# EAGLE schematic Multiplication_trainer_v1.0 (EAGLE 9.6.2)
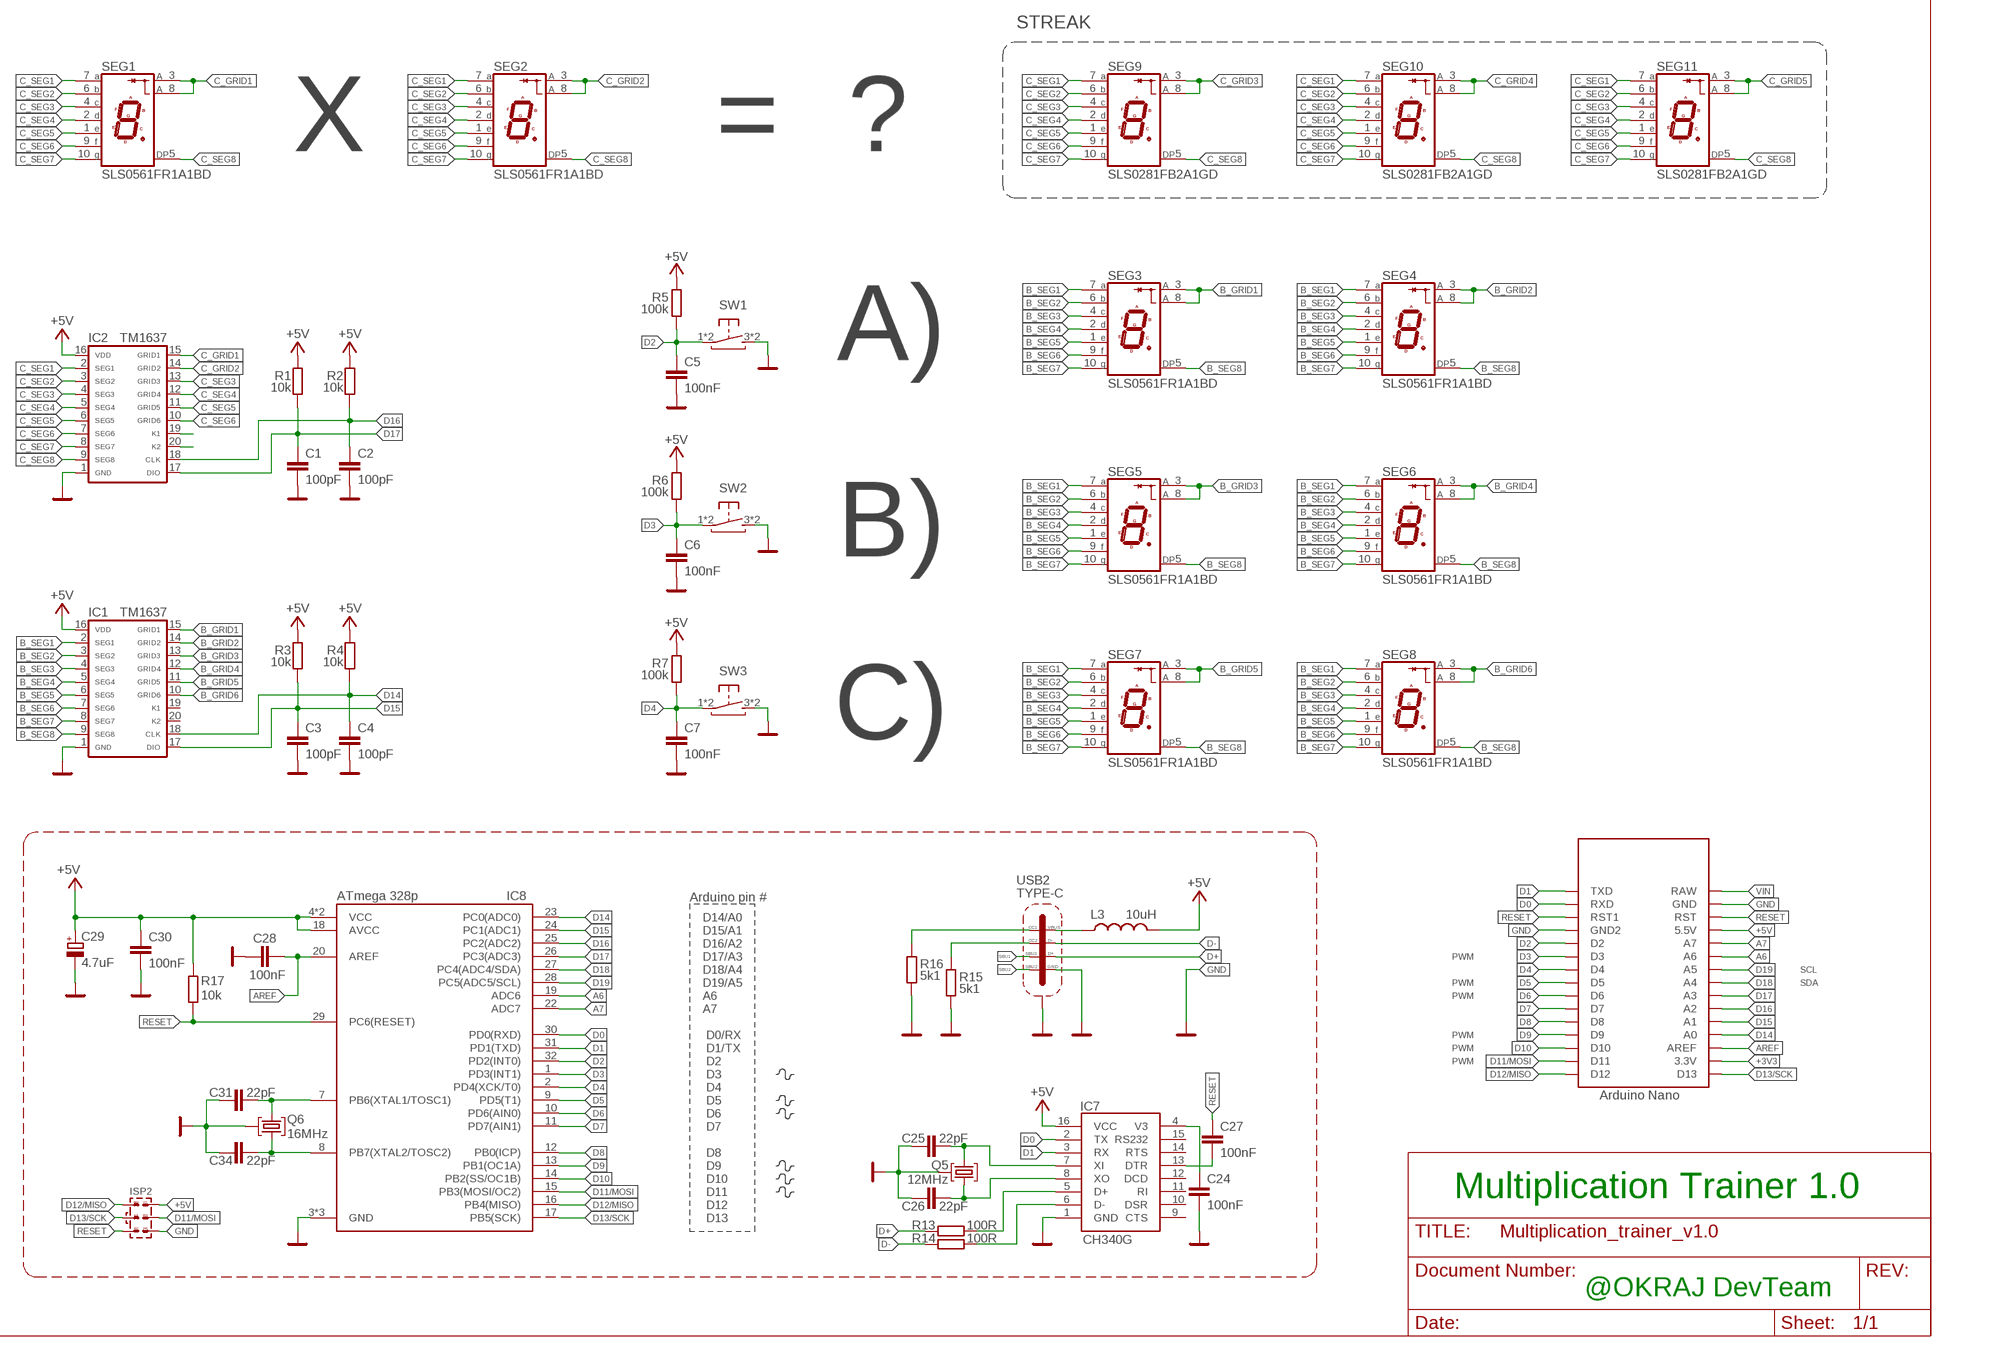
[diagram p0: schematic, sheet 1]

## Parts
C1  100pF  C-EUC0805K  [C0805K]
C2  100pF  C-EUC0805K  [C0805K]
C3  100pF  C-EUC0805K  [C0805K]
C4  100pF  C-EUC0805K  [C0805K]
C5  100nF  C-EUC0805  [C0805]
C6  100nF  C-EUC0805  [C0805]
C7  100nF  C-EUC0805  [C0805]
C24  100nF  C-EUC0603  [C0603]
C25  22pF  C-EUC0603  [C0603]
C26  22pF  C-EUC0603  [C0603]
C27  100nF  C-EUC0603  [C0603]
C28  100nF  C-EUC0603  [C0603]
C29  4.7uF  CPOL-EUSMCA  [SMC_A]
C30  100nF  C-EUC0603  [C0603]
C31  22pF  C-EUC0603  [C0603]
C34  22pF  C-EUC0603  [C0603]
IC1  TM1637  [SOP20]
IC2  TM1637  [SOP20]
IC7  CH340G  CH340GSMD  [SOIC16]
IC8  ATmega 328p  ATMEGA328PQFP32N_ROUND-PADS  [QFP80P900X900X120-32N_ROUND-PADS]
ISP2  AVR-ISP-SPI  [AVR-ISP-SPI]
L3  10uH  L-USL0805  [R0805]
Q5  12MHz  KRYSTAL  [ILCX13-FF5F18-16.0000]
Q6  16MHz  KRYSTAL  [ILCX13-FF5F18-16.0000]
R1  10k  R-EU_R0805  [R0805]
R2  10k  R-EU_R0805  [R0805]
R3  10k  R-EU_R0805  [R0805]
R4  10k  R-EU_R0805  [R0805]
R5  100k  R-EU_R0805  [R0805]
R6  100k  R-EU_R0805  [R0805]
R7  100k  R-EU_R0805  [R0805]
R13  100R  R-EU_R0603  [R0603]
R14  100R  R-EU_R0603  [R0603]
R15  5k1  R-EU_R0603  [R0603]
R16  5k1  R-EU_R0603  [R0603]
R17  10k  R-EU_R0603  [R0603]
SEG1  SLS0561FR1A1BD  [SLS0561FR1A1BD]
SEG2  SLS0561FR1A1BD  [SLS0561FR1A1BD]
SEG3  SLS0561FR1A1BD  [SLS0561FR1A1BD]
SEG4  SLS0561FR1A1BD  [SLS0561FR1A1BD]
SEG5  SLS0561FR1A1BD  [SLS0561FR1A1BD]
SEG6  SLS0561FR1A1BD  [SLS0561FR1A1BD]
SEG7  SLS0561FR1A1BD  [SLS0561FR1A1BD]
SEG8  SLS0561FR1A1BD  [SLS0561FR1A1BD]
SEG9  SLS0281FB2A1GD  [SLS0281FB2A1GD]
SEG10  SLS0281FB2A1GD  [SLS0281FB2A1GD]
SEG11  SLS0281FB2A1GD  [SLS0281FB2A1GD]
SW1  TACT-SW_BTNSMTJLC_6X6X4.5  [TACTSW_6X6X4.5_SMT]
SW2  TACT-SW_BTNSMTJLC_6X6X4.5  [TACTSW_6X6X4.5_SMT]
SW3  TACT-SW_BTNSMTJLC_6X6X4.5  [TACTSW_6X6X4.5_SMT]
U$2  NANOTHT-NOUSB  [NANO-NOUSB]
USB2  TYPE-C  TYPE-C-31-M-12TYPE-C-31_L8.94_W7.3  [TYPE-C-31_L8.94_W7.3]

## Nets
+3V3: U$2.3.3V
+5V: C29.+ C30.1 IC1.16(VDD) IC2.16(VDD) IC7.16(VCC) IC8.4(VCC) IC8.6(VCC) IC8.18(AVCC) ISP2.2 L3.2 R1.2 R2.2 R3.2 R4.2 R5.1 R6.1 R7.1 R17.1 U$2.5V(5.5V)
A6: IC8.19(ADC6) U$2.A6
A7: IC8.22(ADC7) U$2.A7
AREF: C28.1 IC8.20(AREF) U$2.AREF
B_GRID1: IC1.15(GRID1) SEG3.3(CA1) SEG3.8(CA2)
B_GRID2: IC1.14(GRID2) SEG4.3(CA1) SEG4.8(CA2)
B_GRID3: IC1.13(GRID3) SEG5.3(CA1) SEG5.8(CA2)
B_GRID4: IC1.12(GRID4) SEG6.3(CA1) SEG6.8(CA2)
B_GRID5: IC1.11(GRID5) SEG7.3(CA1) SEG7.8(CA2)
B_GRID6: IC1.10(GRID6) SEG8.3(CA1) SEG8.8(CA2)
B_SEG1: IC1.2(SEG1) SEG3.7(A) SEG4.7(A) SEG5.7(A) SEG6.7(A) SEG7.7(A) SEG8.7(A)
B_SEG2: IC1.3(SEG2) SEG3.6(B) SEG4.6(B) SEG5.6(B) SEG6.6(B) SEG7.6(B) SEG8.6(B)
B_SEG3: IC1.4(SEG3) SEG3.4(C) SEG4.4(C) SEG5.4(C) SEG6.4(C) SEG7.4(C) SEG8.4(C)
B_SEG4: IC1.5(SEG4) SEG3.2(D) SEG4.2(D) SEG5.2(D) SEG6.2(D) SEG7.2(D) SEG8.2(D)
B_SEG5: IC1.6(SEG5) SEG3.1(E) SEG4.1(E) SEG5.1(E) SEG6.1(E) SEG7.1(E) SEG8.1(E)
B_SEG6: IC1.7(SEG6) SEG3.9(F) SEG4.9(F) SEG5.9(F) SEG6.9(F) SEG7.9(F) SEG8.9(F)
B_SEG7: IC1.8(SEG7) SEG3.10(G) SEG4.10(G) SEG5.10(G) SEG6.10(G) SEG7.10(G) SEG8.10(G)
B_SEG8: IC1.9(SEG8) SEG3.5(DP) SEG4.5(DP) SEG5.5(DP) SEG6.5(DP) SEG7.5(DP) SEG8.5(DP)
C_GRID1: IC2.15(GRID1) SEG1.3(CA1) SEG1.8(CA2)
C_GRID2: IC2.14(GRID2) SEG2.3(CA1) SEG2.8(CA2)
C_GRID3: SEG9.3(CA1) SEG9.8(CA2)
C_GRID4: SEG10.3(CA1) SEG10.8(CA2)
C_GRID5: SEG11.3(CA1) SEG11.8(CA2)
C_SEG1: IC2.2(SEG1) SEG1.7(A) SEG2.7(A) SEG9.7(A) SEG10.7(A) SEG11.7(A)
C_SEG2: IC2.3(SEG2) SEG1.6(B) SEG2.6(B) SEG9.6(B) SEG10.6(B) SEG11.6(B)
C_SEG3: IC2.4(SEG3) IC2.13(GRID3) SEG1.4(C) SEG2.4(C) SEG9.4(C) SEG10.4(C) SEG11.4(C)
C_SEG4: IC2.5(SEG4) IC2.12(GRID4) SEG1.2(D) SEG2.2(D) SEG9.2(D) SEG10.2(D) SEG11.2(D)
C_SEG5: IC2.6(SEG5) IC2.11(GRID5) SEG1.1(E) SEG2.1(E) SEG9.1(E) SEG10.1(E) SEG11.1(E)
C_SEG6: IC2.7(SEG6) IC2.10(GRID6) SEG1.9(F) SEG2.9(F) SEG9.9(F) SEG10.9(F) SEG11.9(F)
C_SEG7: IC2.8(SEG7) SEG1.10(G) SEG2.10(G) SEG9.10(G) SEG10.10(G) SEG11.10(G)
C_SEG8: IC2.9(SEG8) SEG1.5(DP) SEG2.5(DP) SEG9.5(DP) SEG10.5(DP) SEG11.5(DP)
D0: IC7.2(TX) IC8.30(PD0(RXD)) U$2.RX1(RXD)
D1: IC7.3(RX) IC8.31(PD1(TXD)) U$2.TX0(TXD)
D2: C5.1 IC8.32(PD2(INT0)) R5.2 SW1.1(P) SW1.2(P) U$2.D2
D3: C6.1 IC8.1(PD3(INT1)) R6.2 SW2.1(P) SW2.2(P) U$2.D3
D4: C7.1 IC8.2(PD4(XCK/T0)) R7.2 SW3.1(P) SW3.2(P) U$2.D4
D5: IC8.9(PD5(T1)) U$2.D5
D6: IC8.10(PD6(AIN0)) U$2.D6
D7: IC8.11(PD7(AIN1)) U$2.D7
D8: IC8.12(PB0(ICP)) U$2.D8
D9: IC8.13(PB1(OC1A)) U$2.D9
D10: IC8.14(PB2(SS/OC1B)) U$2.D10
D11/MOSI: IC8.15(PB3(MOSI/OC2)) ISP2.4 U$2.D11
D12/MISO: IC8.16(PB4(MISO)) ISP2.1 U$2.D12
D13/SCK: IC8.17(PB5(SCK)) ISP2.3 U$2.D13
D14: C4.1 IC1.18(CLK) IC8.23(PC0(ADC0)) R4.1 U$2.A0
D15: C3.1 IC1.17(DIO) IC8.24(PC1(ADC1)) R3.1 U$2.A1
D16: C2.1 IC2.18(CLK) IC8.25(PC2(ADC2)) R2.1 U$2.A2
D17: C1.1 IC2.17(DIO) IC8.26(PC3(ADC3)) R1.1 U$2.A3
D18: IC8.27(PC4(ADC4/SDA)) U$2.A4
D19: IC8.28(PC5(ADC5/SCL)) U$2.A5
D+: R13.1 USB2.A6(D+) USB2.B6(D+)
D-: R14.1 USB2.A7(D-) USB2.B7(D-)
GND: C1.2 C2.2 C3.2 C4.2 C5.2 C6.2 C7.2 C24.2 C25.2 C26.2 C28.2 C29.- C30.2 C31.2 C34.2 IC1.1(GND) IC2.1(GND) IC7.1(GND) IC8.3(GND) IC8.5(GND) IC8.21(GND) ISP2.6 Q5.P$2(GND) Q5.P$4(GND) Q6.P$2(GND) Q6.P$4(GND) R15.1 R16.1 SW1.3(S) SW1.4(S) SW2.3(S) SW2.4(S) SW3.3(S) SW3.4(S) U$2.GND U$2.GND1(GND2) USB2.A1/B12(GND) USB2.B1/A12(GND) USB2.SHIELD1(SHIELD) USB2.SHIELD2(SHIELD) USB2.SHIELD3(SHIELD) USB2.SHIELD4(SHIELD) USB2.SHIELD5(SHIELD) USB2.SHIELD6(SHIELD) USB2.SHIELD7(SHIELD) USB2.SHIELD8(SHIELD)
N$6: IC2.19(K1)
N$7: IC2.20(K2)
N$18: C24.1 IC7.4(V3)
N$19: C25.1 IC7.7(XI) Q5.P$1
N$20: C26.1 IC7.8(XO) Q5.P$3
N$27: C27.2 IC7.13(DTR)
N$28: IC7.5(D+) R13.2
N$30: IC7.6(D-) R14.2
N$31: L3.1 USB2.A4/B9(VBUS) USB2.B4/A9(VBUS)
N$32: R15.2 USB2.B5(CC2)
N$33: R16.2 USB2.A5(CC1)
N$34: C31.1 IC8.7(PB6(XTAL1/TOSC1)) Q6.P$1
N$35: C34.1 IC8.8(PB7(XTAL2/TOSC2)) Q6.P$3
RESET: C27.1 IC8.29(PC6(RESET)) ISP2.5 R17.2 U$2.RST U$2.RST1
SBU1: USB2.A8(SBU1)
SBU2: USB2.B8(SBU2)
VIN: U$2.RAW
Unconnected: IC1.19(K1) IC1.20(K2) IC7.9(CTS) IC7.10(DSR) IC7.11(RI) IC7.12(DCD) IC7.14(RTS) IC7.15(RS232)

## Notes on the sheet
- STREAK
- X | = | ?
- A)
- B)
- C)
- Arduino pin #
- D14/A0
- D15/A1
- D16/A2
- D17/A3 | PWM
- D18/A4 | SCL
- D19/A5 | PWM | SDA
- A6 | PWM
- A7
- D0/RX | PWM
- D1/TX | PWM
- D2 | PWM
- D3
- D4
- D5
- D6
- D7
- D8
- D9
- D10
- D11
- Multiplication Trainer 1.0
- D12
- D13
- @OKRAJ DevTeam

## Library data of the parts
C1-C4 = rcl:C-EU: CAPACITOR, European symbol; LCSC_PART: C1790; SPICEPREFIX: C
C5-C7 = rcl:C-EU: CAPACITOR, European symbol
C24 C27 C28 C30 = rcl:C-EU: CAPACITOR, European symbol; LCSC_PART: C49678; SPICEPREFIX: C
C25 C26 C31 C34 = rcl:C-EU: CAPACITOR, European symbol; LCSC_PART: C1804; SPICEPREFIX: C
C29 = rcl:CPOL-EU: POLARIZED CAPACITOR, European symbol; LCSC_PART: C111040; ROT: 180; SPICEPREFIX: C
IC1 IC2 = #my:TM1637; LCSC_PART: C20001; ROT: 270
IC7 = ch340g:CH340G; LCSC_PART: C14267
IC8 = ATMEGA328P-ANR:ATMEGA328P: 8-bit Microcontrollers - MCU AVR 32K FLSH 2K SRAM 1KB EE-20 MHZ 105C Source: Datasheet; LCSC_PART: C14877; ROT: 270
ISP2 = #Ondra2:AVR-ISP-SPI
L3 = rcl:L-US: INDUCTOR, American symbol; LCSC_PART: C281113
Q5 = #Marek:KRYSTAL: Monolithic Crystal Filters Source: www.vanlong.com; LCSC_PART: C9002
Q6 = #Marek:KRYSTAL: Monolithic Crystal Filters Source: www.vanlong.com; LCSC_PART: C13738
R1-R4 R13 R14 R17 = rcl:R-EU_: RESISTOR, European symbol; SPICEPREFIX: R
R5-R7 = resistor:R-EU_: RESISTOR, European symbol
R15 R16 = rcl:R-EU_: RESISTOR, European symbol; LCSC_PART: C27834; SPICEPREFIX: R
SEG1-SEG8 = #my:SLS0561FR1A1BD; LCSC_PART: C226002
SEG9-SEG11 = #my:SLS0281FB2A1GD; LCSC_PART: C225995
SW1-SW3 = #Ondra2:TACT-SW_BTN; LCSC_PART: C127509
U$2 = Arduino-clone:NANO: Arduino Nano
USB2 = #Marek:TYPE-C-31-M-12; LCSC_PART: C165948; ROT: 180

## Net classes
0 default: width 0.127 mm, drill 0.2 mm, clearance 0.127 mm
